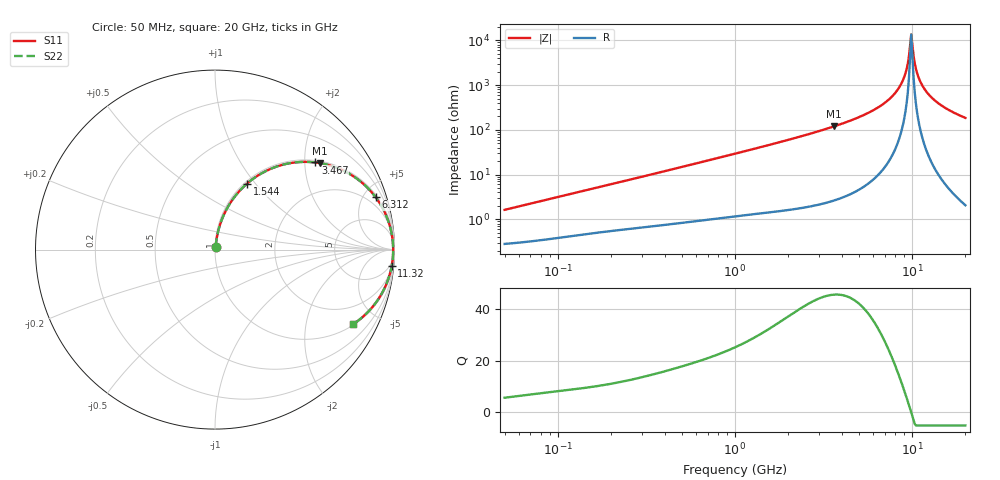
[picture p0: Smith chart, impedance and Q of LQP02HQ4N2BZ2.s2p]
!Murata Part Number: LQP02HQ4N2BZ2
!These Parameters are Measured in Series Mode Connection
!  o--[Z]--o
!Port1  Port2
!  o-------o
!Freq. Start=50[MHz] Stop=20[GHz], 401[Steps]
# Hz S RI R 50
!Freq.(Hz) S11(Real) S11(Imag) S21(Real) S21(Imag) S12(Real) S12(Imag) S22(Real) S22(Imag)
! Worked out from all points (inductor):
!   401 points, 50 MHz to 20 GHz, reference 50 ohm
!   read as one part in series: L = 5.06 nH near 51.52 MHz
!   highest Q = 45.5 at 3.626 GHz (marker M1), where L = 5.25 nH
!   self-resonance near 9.892 GHz
!   S11 on the Smith chart (normalised r, x): 50 MHz: 1.01, +0.03; 1.544 GHz: 1.03, +0.91; 3.467 GHz: 1.05, +2.26; 6.312 GHz: 1.18, +6.06; 11.32 GHz: 3, -21; 20 GHz: 1.04, -3.70
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5e7  0.00306 0.0159  0.9969 -0.0159  0.9969 -0.0159  0.00306 0.0159
1.364002e8  0.00624 0.0417  0.9938 -0.0417  0.9938 -0.0417  0.00624 0.0417
3.721004e8  0.019 0.1075  0.981 -0.1075  0.981 -0.1075  0.019 0.1075
1e9  0.0876 0.2636  0.9124 -0.2636  0.9124 -0.2636  0.0876 0.2636
1.544007e9  0.1789 0.368  0.8211 -0.368  0.8211 -0.368  0.1789 0.368
2.728004e9  0.4178 0.4816  0.5822 -0.4816  0.5822 -0.4816  0.4178 0.4816
3.466789e9  0.5587 0.4856  0.4413 -0.4856  0.4413 -0.4856  0.5587 0.4856
3.626126e9  0.5865 0.4816  0.4135 -0.4816  0.4135 -0.4816  0.5865 0.4816
4.966507e9  0.7764 0.405  0.2236 -0.405  0.2236 -0.405  0.7764 0.405
6.311513e9  0.8948 0.2921  0.1052 -0.2921  0.1052 -0.2921  0.8948 0.2921
7.442007e9  0.9521 0.1934  0.0479 -0.1934  0.0479 -0.1934  0.9521 0.1934
8.264682e9  0.9761 0.1245  0.0239 -0.1245  0.0239 -0.1245  0.9761 0.1245
8.907419e9  0.9868 0.0734  0.0132 -0.0734  0.0132 -0.0734  0.9868 0.0734
9.316812e9  0.9907 0.0422  0.00932 -0.0422  0.00932 -0.0422  0.9907 0.0422
9.745021e9  0.9925 0.0109  0.00747 -0.0109  0.00747 -0.0109  0.9925 0.0109
9.892087e9  0.9927 0.000448  0.0073 -0.000448  0.0073 -0.000448  0.9927 0.000448
1.019291e10  0.9924 -0.0205  0.00762 0.0205  0.00762 0.0205  0.9924 -0.0205
1.066139e10  0.9902 -0.0518  0.00977 0.0518  0.00977 0.0518  0.9902 -0.0518
1.131968e10  0.9843 -0.0932  0.0157 0.0932  0.0157 0.0932  0.9843 -0.0932
1.238412e10  0.9688 -0.1541  0.0312 0.1541  0.0312 0.1541  0.9688 -0.1541
1.396067e10  0.9364 -0.2313  0.0636 0.2313  0.0636 0.2313  0.9364 -0.2313
2e10  0.7712 -0.4146  0.2288 0.4146  0.2288 0.4146  0.7712 -0.4146
